FUNCTION_BLOCK FB_PushPopStack  //队列功能块，用于HMI中存储显示Nci指令
VAR_IN_OUT
	ArrayNciCommand: ARRAY[1..100] OF Nci_SingleEntry;
END_VAR
VAR_INPUT
	PushCommand:  Nci_SingleEntry;
END_VAR
VAR_OUTPUT
	PopCommand	: Nci_SingleEntry;
	busy						: BOOL;
END_VAR
VAR
	i: INT;
END_VAR

;

METHOD ClearStack : BOOL //清空队列
VAR_INPUT
END_VAR
busy:=TRUE;
FOR i:=1 TO 100 DO
	ArrayNciCommand[i].SyncVelo:=0;
    ArrayNciCommand[i].SyncAcc:=0;
    ArrayNciCommand[i].fX:=0;
    ArrayNciCommand[i].fY:=0;
    ArrayNciCommand[i].fZ:=0;
    ArrayNciCommand[i].fQ1:=0;
    ArrayNciCommand[i].fQ2:=0;
    ArrayNciCommand[i].fQ3:=0;
    ArrayNciCommand[i].fQ4:=0;
    ArrayNciCommand[i].fQ5:=0;
    ArrayNciCommand[i].fCenterX:=0;
    ArrayNciCommand[i].fCenterY:=0;
    ArrayNciCommand[i].fCenterZ:=0;
    ArrayNciCommand[i].bClockwise:=FALSE;
    ArrayNciCommand[i].iPlane:=0;
END_FOR
END_METHOD

METHOD PopStack : BOOL //提取队列数据
VAR_INPUT
END_VAR

VAR
	i: INT;
END_VAR
busy:=TRUE;
PopCommand:=ArrayNciCommand[1];
FOR i:=2 TO 100 DO
	ArrayNciCommand[i-1]:=ArrayNciCommand[i];
END_FOR
ArrayNciCommand[100].SyncVelo:=0;
ArrayNciCommand[100].SyncAcc:=0;
ArrayNciCommand[100].fX:=0;
ArrayNciCommand[100].fY:=0;
ArrayNciCommand[100].fZ:=0;
ArrayNciCommand[100].fQ1:=0;
ArrayNciCommand[100].fQ2:=0;
ArrayNciCommand[100].fQ3:=0;
ArrayNciCommand[100].fQ4:=0;
ArrayNciCommand[100].fQ5:=0;
ArrayNciCommand[100].fCenterX:=0;
ArrayNciCommand[100].fCenterY:=0;
ArrayNciCommand[100].fCenterZ:=0;
ArrayNciCommand[100].bClockwise:=FALSE;
ArrayNciCommand[100].iPlane:=0;
busy:=FALSE;
END_METHOD

METHOD PushStack : BOOL//存储队列数据
VAR_INPUT
END_VAR
busy:=TRUE;
FOR i:=1 TO 100 DO
	IF ArrayNciCommand[i].SyncVelo=0 THEN
		ArrayNciCommand[i]:=PushCommand;
		EXIT;
	END_IF
END_FOR
busy:=FALSE;
END_METHOD

END_FUNCTION_BLOCK
